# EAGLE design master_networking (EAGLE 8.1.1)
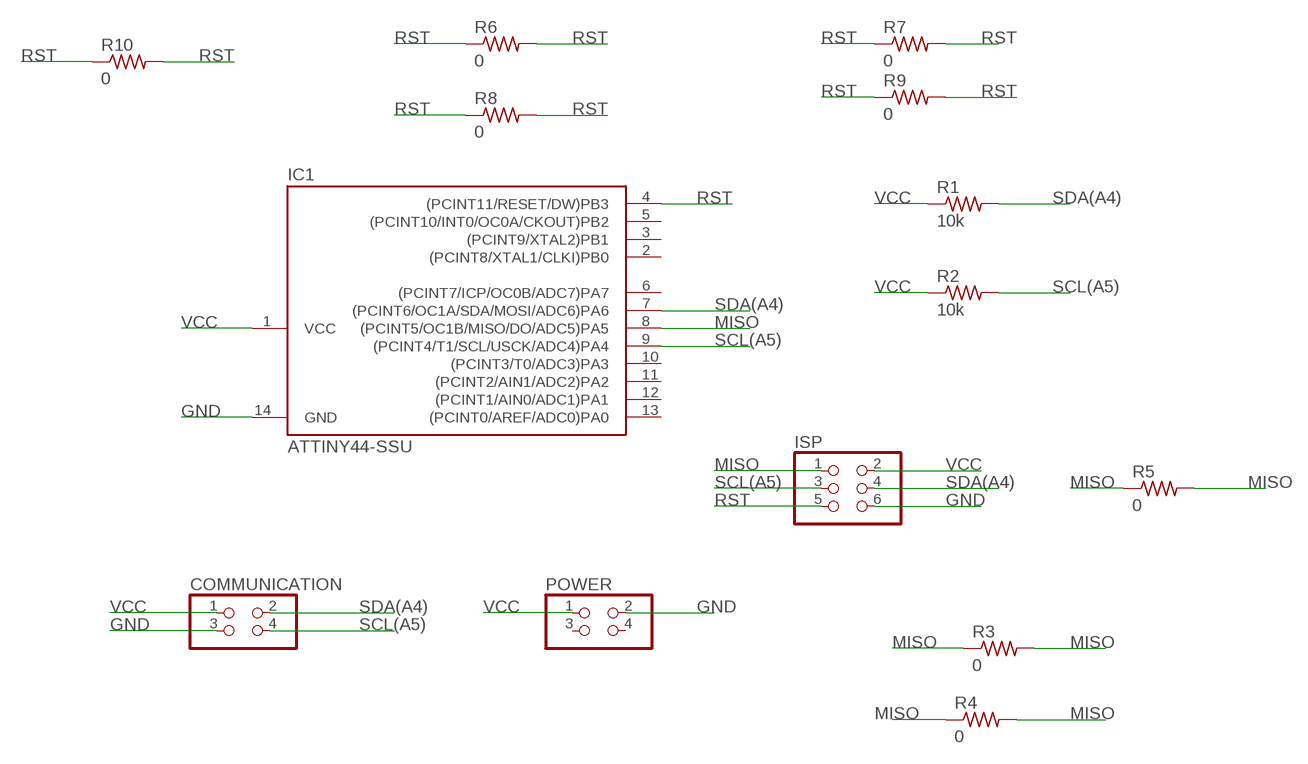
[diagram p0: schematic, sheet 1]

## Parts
COMMUNICATION  PINHD-2X2-SMD  [2X02SMD]
IC1  ATTINY44-SSU  [SOIC14]
ISP  PINHD-2X3-SMD  [2X03SMD]
POWER  PINHD-2X2-SMD  [2X02SMD]
R1  10k  RES-US1206FAB  [R1206FAB]
R2  10k  RES-US1206FAB  [R1206FAB]
R3  0  RES-US1206FAB  [R1206FAB]
R4  0  RES-US1206FAB  [R1206FAB]
R5  0  RES-US1206FAB  [R1206FAB]
R6  0  RES-US1206FAB  [R1206FAB]
R7  0  RES-US1206FAB  [R1206FAB]
R8  0  RES-US1206FAB  [R1206FAB]
R9  0  RES-US1206FAB  [R1206FAB]
R10  0  RES-US1206FAB  [R1206FAB]

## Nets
GND: COMMUNICATION.3 IC1.14(GND) ISP.6 POWER.2
MISO: IC1.8((PCINT5/OC1B/MISO/DO/ADC5)PA5) ISP.1 R3.1 R3.2 R4.1 R4.2 R5.1 R5.2
RST: IC1.4((PCINT11/RESET/DW)PB3) ISP.5 R6.1 R6.2 R7.1 R7.2 R8.1 R8.2 R9.1 R9.2 R10.1 R10.2
SCL(A5): COMMUNICATION.4 IC1.9((PCINT4/T1/SCL/USCK/ADC4)PA4) ISP.3 R2.2
SDA(A4): COMMUNICATION.2 IC1.7((PCINT6/OC1A/SDA/MOSI/ADC6)PA6) ISP.4 R1.2
VCC: COMMUNICATION.1 IC1.1(VCC) ISP.2 POWER.1 R1.1 R2.1
Unconnected: IC1.2((PCINT8/XTAL1/CLKI)PB0) IC1.3((PCINT9/XTAL2)PB1) IC1.5((PCINT10/INT0/OC0A/CKOUT)PB2) IC1.6((PCINT7/ICP/OC0B/ADC7)PA7) IC1.10((PCINT3/T0/ADC3)PA3) IC1.11((PCINT2/AIN1/ADC2)PA2) IC1.12((PCINT1/AIN0/ADC1)PA1) IC1.13((PCINT0/AREF/ADC0)PA0) POWER.3 POWER.4

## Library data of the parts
COMMUNICATION POWER = fab:PINHD-2X2-SMD
IC1 = fab:ATTINY44
ISP = fab:PINHD-2X3-SMD: PIN HEADER
R1-R10 = fab:RES-US: Resistor (US Symbol)

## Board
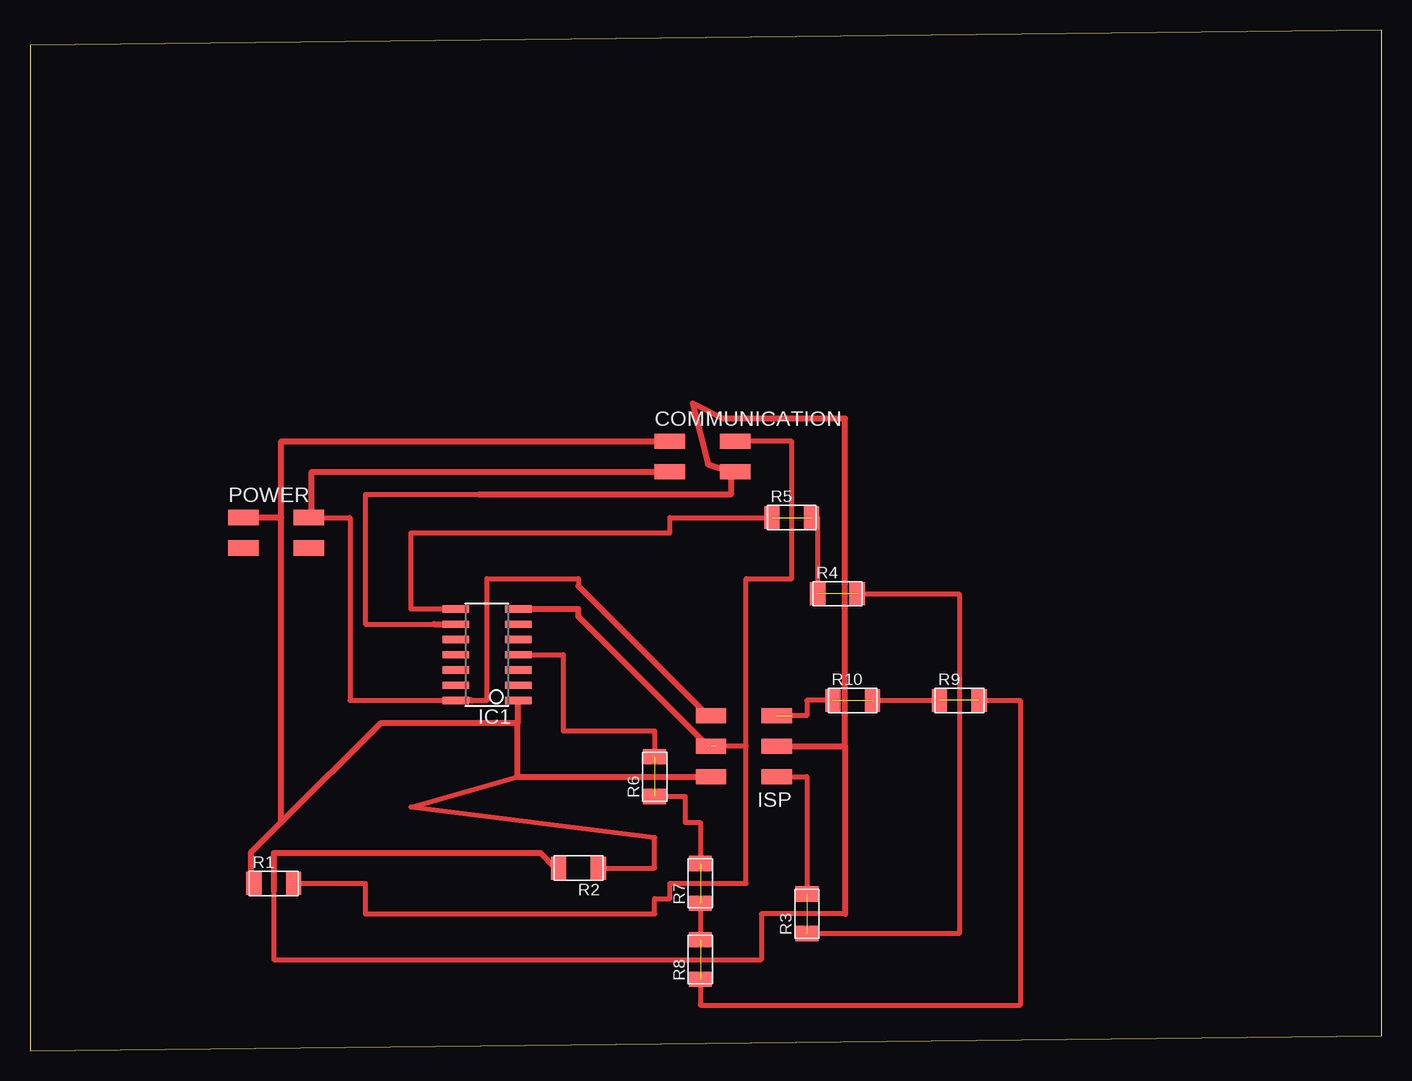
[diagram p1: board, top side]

Size 112.7 x 85.08 mm. Coordinates in mm from the lower left corner, seen from the top.
Outline: 0,0 112.7,1.27 112.7,85.08 0,83.81 0,0
Copper layers (1*16): Top 0.035mm / dielectric 1.5mm / Bottom 0.035mm
Design rules "default *": minimum track width 20mil, minimum drill 24mil, track to track 32mil, track to pad 8mil, pad to pad 8mil, via to via 8mil, smd to smd 8mil, copper to edge 40mil, drill to drill 8mil, minimum pad ring 10mil, minimum via ring 8mil, stop-mask expansion 4mil, vias tented up to drill 0mil, thermal gap 10mil

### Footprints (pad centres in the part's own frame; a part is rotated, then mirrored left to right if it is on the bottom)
2X02SMD = smd 2.54 x 1.27: 1 -2.54,1.27; 2 2.92,1.27; 3 -2.54,-1.27; 4 2.92,-1.27
SOIC14 = smd 0.61 x 2.21: 1 -3.81,-2.603; 2 -2.54,-2.603; 3 -1.27,-2.603; 4 0,-2.603; 5 1.27,-2.603; 6 2.54,-2.603; 7 3.81,-2.603; 8 3.81,2.603; 9 2.54,2.603; 10 1.27,2.603; 11 0,2.603; 12 -1.27,2.603; 13 -2.54,2.603; 14 -3.81,2.603
2X03SMD = smd 2.54 x 1.27: 1 -2.54,2.54; 2 2.92,2.54; 3 -2.54,0; 4 2.92,0; 5 -2.54,-2.54; 6 2.92,-2.54
R1206FAB = smd 1.27 x 1.905: 1 -1.651,0; 2 1.651,0

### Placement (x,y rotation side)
COMMUNICATION  55.88,49.53 0 top
IC1  38.1,33.02 90 top
ISP  59.69,25.4 180 top
POWER  20.32,43.18 0 top
R1  20.32,13.97 0 top
R2  45.72,15.24 180 top
R3  64.77,11.43 90 top
R4  67.31,38.1 0 top
R5  63.5,44.45 0 top
R6  52.07,22.86 90 top
R7  55.88,13.97 90 top
R8  55.88,7.62 90 top
R9  77.47,29.21 0 top
R10  68.58,29.21 0 top

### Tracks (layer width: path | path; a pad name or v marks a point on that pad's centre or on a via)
GND
  Top 0.406: POWER.2 26.67,44.45 26.67,29.21 IC1.14 38.1,29.21 38.1,39.37 45.72,39.37 45.72,38.73
  Top 0.508: COMMUNICATION.3 23.49,48.26 23.49,44.45 POWER.2 | 45.72,38.73 56.52,27.94 ISP.6 | 36.83,29.21 IC1.14
MISO  (3 unrouted)
  Top 0.406: ISP.1 64.77,22.86 R3.2 | R3.1 77.47,9.78 77.47,38.1 R4.2 | R5.2 65.66,44.45 R4.1 | IC1.8 31.75,36.83 31.75,43.18 53.34,43.18 53.34,44.45 R5.1
RST  (6 unrouted)
  Top 0.406: R6.1 54.61,21.21 54.61,19.05 55.88,19.05 R7.2 | R8.1 55.88,3.81 82.55,3.81 82.55,29.21 R9.2 | R10.2 R9.1 | R10.1 64.77,29.21 64.77,27.94 63.5,27.94 | IC1.4 44.45,33.02 44.45,26.67 52.07,26.67 R6.2 | R7.1 R8.2
SCL(A5)
  Top 0.406: 38.1,46.35 27.94,46.35 27.94,35.56 33.66,35.56 | 67.94,11.43 60.96,11.43 60.96,7.62 20.32,7.62 20.32,13.34
  Top 0.508: 33.66,35.56 IC1.9 | 37.47,46.35 38.1,46.35 58.42,46.35 58.42,48.26 | 20.32,13.34 20.32,16.51 42.55,16.51 43.81,15.24 R2.2 | 67.94,25.4 67.94,11.43 | ISP.3 67.94,25.4 | 58.42,48.26 56.52,48.89 55.25,53.98 57.78,52.7 67.94,52.7 67.94,25.4 | 58.42,48.26 COMMUNICATION.4
SDA(A4)  (1 unrouted)
  Top 0.406: R1.2 27.94,13.97 27.94,11.43 52.07,11.43 52.07,12.7 53.34,12.7 53.34,13.97 59.69,13.97 59.69,25.4 | 59.69,25.4 57.15,25.4 | 59.69,25.4 59.69,39.37 63.5,39.37 63.5,50.8 COMMUNICATION.2
  Top 0.508: IC1.7 45.72,36.83 45.72,36.2 56.52,25.4 ISP.4
VCC
  Top 0.406: R2.1 52.07,15.24 52.07,17.78 31.75,20.32 40.64,22.86
  Top 0.508: 20.95,19.05 29.21,27.3 40.64,27.3 | 20.95,19.05 18.41,16.51 18.41,13.97 R1.1 | 40.64,27.3 40.64,29.21 IC1.1 | 40.64,27.3 40.64,22.86 ISP.2 | 20.95,44.45 POWER.1 | 20.95,19.05 20.95,44.45 | COMMUNICATION.1 20.95,50.8 20.95,44.45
